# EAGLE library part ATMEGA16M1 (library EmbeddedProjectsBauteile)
Atmel Low Power AVR 8-bit Microcontroller 16K with CAN
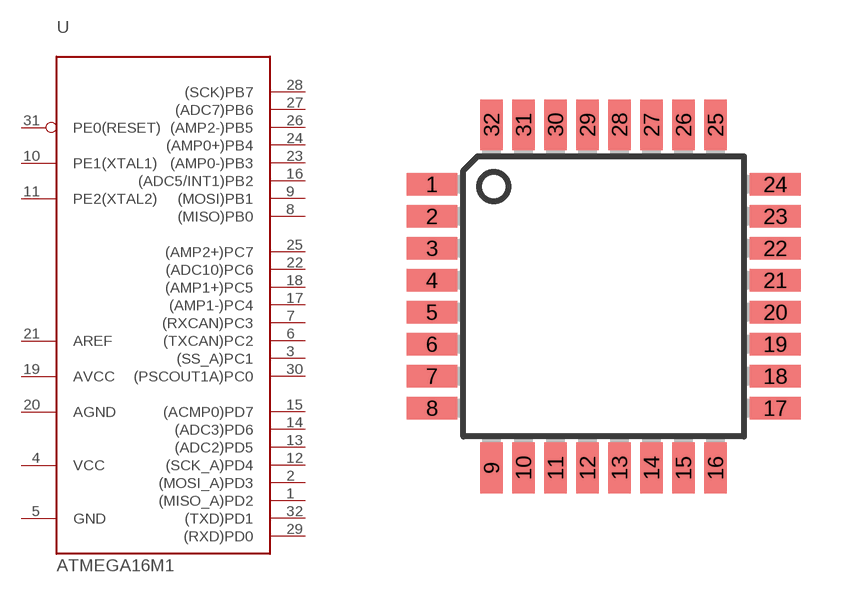
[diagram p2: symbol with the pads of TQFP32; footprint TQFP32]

Designator prefix -

## ATMEGA16M1 (EP: 40880)  [TQFP32]
1  (MISO_A)PD2
2  (MOSI_A)PD3
3  (SS_A)PC1
4  VCC  pwr
5  GND  pwr
6  (TXCAN)PC2
7  (RXCAN)PC3
8  (MISO)PB0
9  (MOSI)PB1
10  PE1(XTAL1)
11  PE2(XTAL2)
12  (SCK_A)PD4
13  (ADC2)PD5
14  (ADC3)PD6
15  (ACMP0)PD7
16  (ADC5/INT1)PB2
17  (AMP1-)PC4
18  (AMP1+)PC5
19  AVCC  pwr
20  AGND  pwr
21  AREF  pas
22  (ADC10)PC6
23  (AMP0-)PB3
24  (AMP0+)PB4
25  (AMP2+)PC7
26  (AMP2-)PB5
27  (ADC7)PB6
28  (SCK)PB7
29  (RXD)PD0
30  (PSCOUT1A)PC0
31  PE0(RESET)  in
32  (TXD)PD1

## Footprint TQFP32 (pad centres in mm)
smd 1.27 x 0.559: 1 -4.293,2.8; 2 -4.293,2; 3 -4.293,1.2; 4 -4.293,0.4; 5 -4.293,-0.4; 6 -4.293,-1.2; 7 -4.293,-2; 8 -4.293,-2.8; 17 4.293,-2.8; 18 4.293,-2; 19 4.293,-1.2; 20 4.293,-0.4; 21 4.293,0.4; 22 4.293,1.2; 23 4.293,2; 24 4.293,2.8
smd 0.559 x 1.27: 9 -2.8,-4.293; 10 -2,-4.293; 11 -1.2,-4.293; 12 -0.4,-4.293; 13 0.4,-4.293; 14 1.2,-4.293; 15 2,-4.293; 16 2.8,-4.293; 25 2.8,4.293; 26 2,4.293; 27 1.2,4.293; 28 0.4,4.293; 29 -0.4,4.293; 30 -1.2,4.293; 31 -2,4.293; 32 -2.8,4.293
